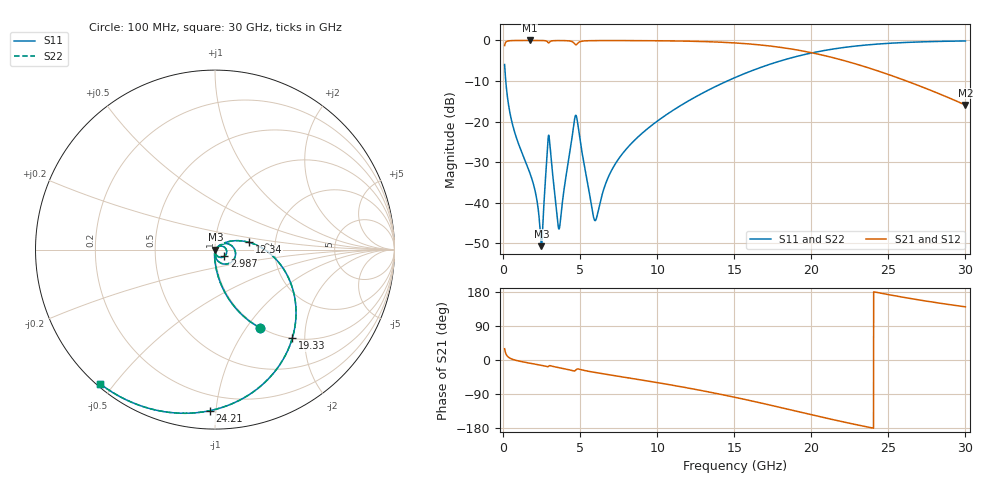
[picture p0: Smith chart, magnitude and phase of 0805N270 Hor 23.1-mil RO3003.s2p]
# GHz S MA R 50
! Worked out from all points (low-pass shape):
!   3201 points, 100 MHz to 30 GHz, reference 50 ohm
!   highest |S21| = -0.01 dB at 1.744 GHz (marker M1); lowest = -15.9 dB at 30 GHz (marker M2)
!   |S21| within 3 dB of the highest: start of sweep to 19.98 GHz
!   lowest |S11| = -50.7 dB at 2.492 GHz (marker M3), VSWR 1.01, Z = 50.3 - j0.12 ohm
!   |S11| at or under -10 dB: 174.7 MHz to 14.55 GHz (14.38 GHz wide, 195 % of centre)
!   |S22| runs from -50.7 to -0.1 dB; largest |S21 - S12| = 0
!   S11 on the Smith chart (normalised r, x): 100 MHz: 0.99, -1.16; 2.987 GHz: 1.11, -0.08; 12.34 GHz: 1.46, +0.12; 19.33 GHz: 1.01, -1.74; 24.21 GHz: 0.10, -0.96; 30 GHz: 0.01, -0.46
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0.1  0.5038 -60.3  0.8634 29.7  0.8634 29.7  0.5038 -60.3
0.62325  0.09028 -87.9  0.9952 1.7  0.9952 1.7  0.09028 -87.9
1.7445  0.02308 -95.3  0.9984 -8.4  0.9984 -8.4  0.02308 -95.3
2.108906  0.01315 -94.1  0.9983 -11.0  0.9983 -11.0  0.01315 -94.1
2.492  0.002905 -24.3  0.9971 -13.8  0.9971 -13.8  0.002905 -24.3
2.604125  0.006595 35.7  0.9957 -14.8  0.9957 -14.8  0.006595 35.7
2.856406  0.0408 28.9  0.9713 -17.6  0.9713 -17.6  0.0408 28.9
2.987219  0.06494 -35.6  0.9387 -15.3  0.9387 -15.3  0.06494 -35.6
3.631937  0.00472 -17.1  0.9952 -20.2  0.9952 -20.2  0.00472 -17.1
4.650406  0.1098 -0.1  0.9021 -28.7  0.9021 -28.7  0.1098 -0.1
4.80925  0.1044 -50.1  0.9051 -23.9  0.9051 -23.9  0.1044 -50.1
5.089563  0.04545 -84.4  0.9753 -25.9  0.9753 -25.9  0.04545 -84.4
5.986562  0.006009 -21.5  0.9939 -33.0  0.9939 -33.0  0.006009 -21.5
7.35075  0.0315 40.3  0.995 -41.9  0.995 -41.9  0.0315 40.3
10.06978  0.1031 27.5  0.9898 -60.0  0.9898 -60.0  0.1031 27.5
12.34031  0.194 12.0  0.9753 -76.5  0.9753 -76.5  0.194 12.0
15.05  0.3482 -9.5  0.9303 -98.5  0.9303 -98.5  0.3482 -9.5
19.32944  0.6536 -48.7  0.7473 -137.9  0.7473 -137.9  0.6536 -48.7
20.03956  0.7011 -55.4  0.7033 -144.7  0.7033 -144.7  0.7011 -55.4
24.20688  0.8983 -91.9  0.4276 178.7  0.4276 178.7  0.8983 -91.9
25.01978  0.9203 -98.2  0.3791 172.4  0.3791 172.4  0.9203 -98.2
30  0.9843 -130.4  0.1596 140.3  0.1596 140.3  0.9843 -130.4
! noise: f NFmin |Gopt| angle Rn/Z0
0.1  0.000522  0.8834  0.8161  0.0009708
3.417  0.01046  0.8102  18.98  0.01118
6.743  0.01316  0.7227  36.88  0.008497
10.06  0.01589  0.6761  53.59  0.007616
13.39  0.02071  0.6795  69.18  0.008611
16.7  0.02712  0.7016  83.65  0.01013
20.03  0.03614  0.7368  97.33  0.01233
23.35  0.04971  0.782  110.5  0.01567
26.67  0.07225  0.8341  123.5  0.02117
30  0.1147  0.888  136.7  0.03104
